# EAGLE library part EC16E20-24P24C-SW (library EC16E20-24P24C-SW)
Specification ; Resolution. 24imp/revol. ; Number of positions. 24 ; Output signal. two phase A and B ; Mechanical durability. 50000 cycles ; Operating voltage. 5V .. Source: Datasheet
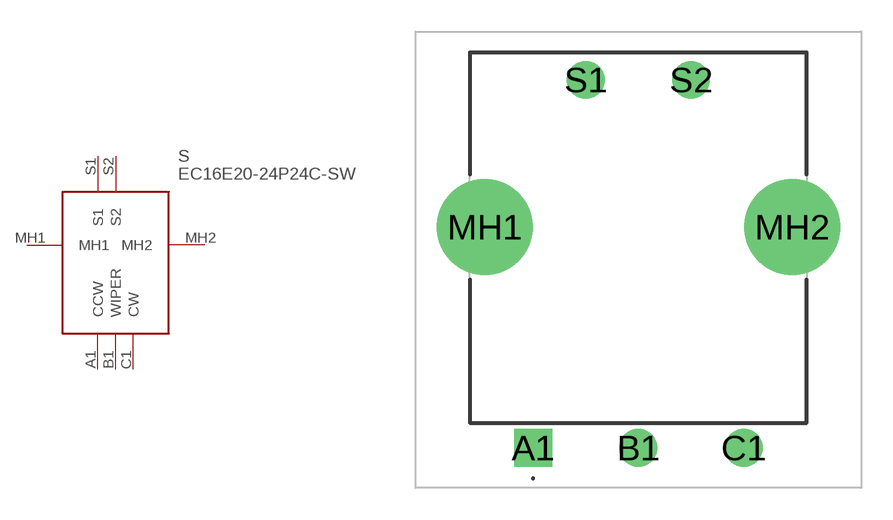
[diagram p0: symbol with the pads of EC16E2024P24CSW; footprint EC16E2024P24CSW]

Designator prefix S

## EC16E20-24P24C-SW (Description: Specification ; Resolution. 24imp/revol. ; Number of positions. 24 ; Output signal. two phase A and B ; Mechanical durability. 50000 cycles ; Operating voltage. 5V ..; Height: 28mm; Manufacturer_Name: SRPASSIVES; Manufacturer_Part_Number: EC16E20-24P24C-SW)  [EC16E2024P24CSW]
A1  CCW
B1  WIPER
C1  CW
MH1  MH1
MH2  MH2
S1  S1
S2  S2

## Footprint EC16E2024P24CSW (pad centres in mm)
EC16E20-24P24C-SW-1
drill 1.2 pad 1.8 square: A1 0,0
drill 1.2 pad 1.8: B1 5,0; C1 10,0; S1 2.5,17.5; S2 7.5,17.5
drill 3.04 pad 4.56: MH1 -2.3,10.5; MH2 12.3,10.5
